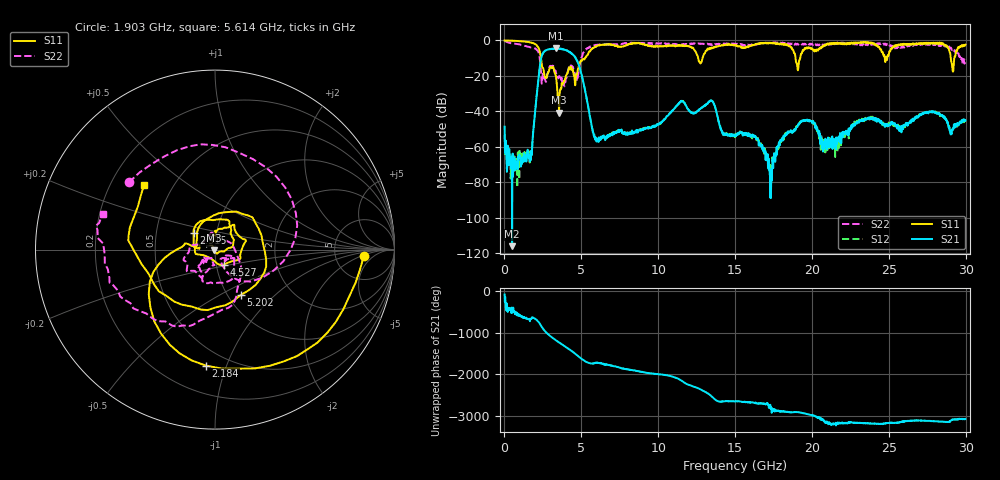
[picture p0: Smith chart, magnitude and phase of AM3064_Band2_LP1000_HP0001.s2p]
# Hz S DB R 50.0
!freq dBS11 angS11 dBS21 angS21 dBS12 angS12 dBS22 angS22
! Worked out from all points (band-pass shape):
!   1600 points, 10 MHz to 29.98 GHz, reference 50 ohm
!   highest |S21| = -4.56 dB at 3.328 GHz (marker M1); lowest = -116.1 dB at 497.3 MHz (marker M2)
!   |S21| within 3 dB of the highest: 2.483 GHz to 4.387 GHz (1.905 GHz wide, 55.5 % of centre)
!   lowest |S11| = -40.8 dB at 3.553 GHz (marker M3), VSWR 1.02, Z = 49.2 - j0.416 ohm
!   |S11| at or under -10 dB: 2.375 GHz to 5.242 GHz (2.867 GHz wide, 75.3 % of centre); 12.6 GHz to 12.88 GHz (283.6 MHz wide, 2.23 % of centre); 18.93 GHz to 19.23 GHz (301.7 MHz wide, 1.58 % of centre)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
!   |S22| runs from -25.9 to -0.2 dB; largest |S21 - S12| = 0.013
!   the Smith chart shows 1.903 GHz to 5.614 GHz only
!   S11 on the Smith chart (normalised r, x): 1.903 GHz: 10, -2; 2.184 GHz: 0.38, -0.85; 2.915 GHz: 0.77, +0.14; 4.527 GHz: 1.09, -0.18; 5.202 GHz: 1.14, -0.63; 5.614 GHz: 0.34, +0.35
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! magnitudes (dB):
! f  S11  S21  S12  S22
! 10 MHz  0.0  -48.6  -53.1  -0.2
! 497.3 MHz  -0.1  -116.1  -65.5  -1.6
! 1.659 GHz  -1.1  -68.3  -62.5  -3.9
! 1.903 GHz  -1.6  -48.7  -48.5  -4.3
! 2.184 GHz  -3.8  -23.7  -23.7  -6.1
! 2.915 GHz  -16.5  -5.0  -4.9  -15.5
! 3.328 GHz  -19.6  -4.6  -4.6  -17.3
! 3.553 GHz  -40.8  -4.8  -4.7  -20.3
! 4.527 GHz  -20.3  -8.6  -8.6  -17.0
! 5.015 GHz  -11.4  -19.3  -19.4  -9.6
! 5.202 GHz  -10.7  -26.5  -26.4  -6.3
! 5.614 GHz  -5.4  -45.5  -45.7  -3.6
! 6.064 GHz  -3.0  -55.7  -56.9  -2.4
! 10 GHz  -3.4  -47.4  -47.1  -1.8
! 13.43 GHz  -4.5  -33.9  -33.9  -2.5
! 15 GHz  -2.6  -54.0  -54.4  -1.8
! 17.33 GHz  -1.3  -88.9  -70.1  -1.4
! 18.29 GHz  -2.3  -53.0  -52.1  -1.9
! 19.99 GHz  -4.6  -46.3  -45.8  -1.9
! 20.85 GHz  -2.7  -56.5  -58.7  -2.6
! 25 GHz  -8.0  -47.5  -46.3  -2.3
! 29.98 GHz  -2.4  -45.1  -45.9  -10.5
